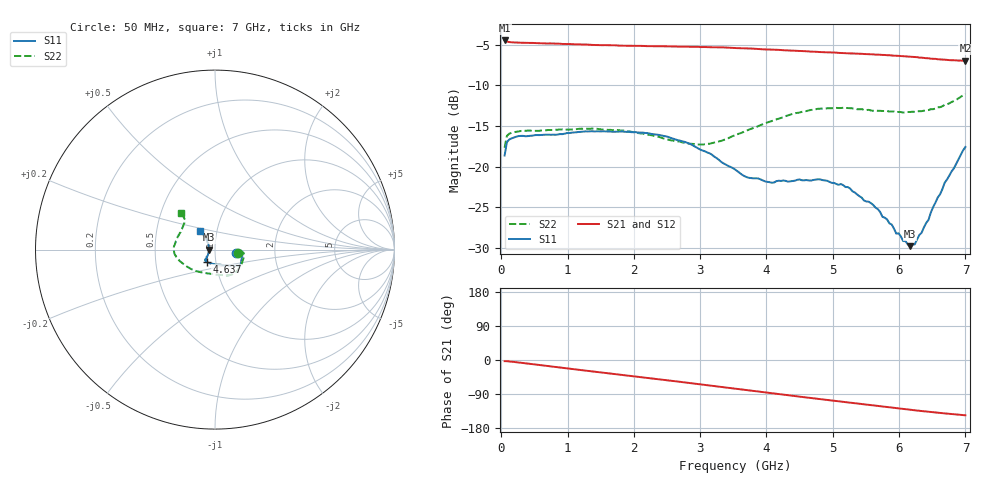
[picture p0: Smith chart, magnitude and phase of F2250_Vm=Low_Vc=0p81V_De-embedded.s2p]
! Integrated Device Technology
! Corporate Headquarters
! 6024 Silver Creek Valley Road
! San Jose, CA 95138  USA
! Phone:  1-408-284-8200
! Toll Free:  1-800-223-1366
! Webpage:  http://www.idt.com/
! Timing and RF Division
! 515 Groton Road, Suite 102
! Westford, MA 01886-6024
! Device:  F2250
! Description: Voltage Variable RF Attenuator
! Frequency:  50.0 -  6000.00 MHz
! Package:  3x3 mm Thin QFN Plastic Package: 16 pin
! Ports:  2 RF, 3 DC
!  Pin  1  = GND
!  Pin  2  = NC
!  Pin  3  = RF1  = Port 1
!  Pin  4  = NC
!  Pin  5  = GND
!  Pin  6  = GND
!  Pin  7  = GND
!  Pin  8  = GND
!  Pin  9  = NC
!  Pin 10  = RF2  = Port 2
!  Pin 11  = NC
!  Pin 12  = GND
!  Pin 13  = GND
!  Pin 14  = VCNTRL
!  Pin 15  = VDD
!  Pin 16  = VMODE
! Vcntrl:  0.810 Volts
! Vmode:  +0.000 Volts
! Vdd:  +3.30  Volts
! Current:  1.166 mA
! Data:  The device was measured on a the F2250 evaluation board which has
!  individual transmission lines to the RF pins.  Data was collected
!  using a calibrated network analyzer.  The evaluation board was
!  de-embedded using a TRL calibration technique.
!  The reference plane is the edge of the package pin.
! Misc:  SN 10
!  Action Tracker AT0258
! Date Measured:  2014-11-26
! Date:  2015-10-15  MJV
! Note:
!  Integrated Device Technology supplies this data as a sample of measured
!  data at the package pin for this product.  Your particular data for this
!  product may vary.
!  Data was taken at 25 degrees C.
!  Integrated Device Technology reserves the right to change this data at anytime.
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# GHz S dB R 50
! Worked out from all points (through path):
!   201 points, 50 MHz to 7 GHz, reference 50 ohm
!   highest |S21| = -4.46 dB at 50 MHz (marker M1); lowest = -7.0 dB at 7 GHz (marker M2)
!   group delay of S21, straight-line fit = 58.5 ps
!   lowest |S11| = -29.8 dB at 6.166 GHz (marker M3), VSWR 1.07, Z = 46.9 - j0.0792 ohm
!   |S11| at or under -10 dB: start of sweep to end of sweep
!   |S22| runs from -17.7 to -11.1 dB; largest |S21 - S12| = 0.0014
!   S11 on the Smith chart (normalised r, x): 50 MHz: 1.26, -0.05; 4.637 GHz: 0.90, -0.12; 7 GHz: 0.83, +0.17
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0.05  -18.64 -8.9  -4.46 -3.0  -4.48 -3.0  -17.67 -8.8
0.08475  -17.00 -5.7  -4.60 -3.2  -4.61 -3.2  -16.22 -6.2
0.22375  -16.32 -6.9  -4.72 -5.7  -4.73 -5.7  -15.72 -9.6
1.2315  -15.70 -27.8  -4.97 -27.2  -4.95 -27.2  -15.33 -43.2
1.857  -15.71 -32.8  -5.12 -40.1  -5.11 -40.1  -15.57 -57.5
2.37825  -16.10 -35.2  -5.17 -50.9  -5.19 -50.9  -16.35 -70.2
3.0385  -18.03 -44.8  -5.28 -65.0  -5.27 -65.0  -17.29 -100.4
3.525  -20.36 -64.6  -5.39 -75.6  -5.41 -75.6  -16.15 -128.5
3.69875  -21.30 -75.4  -5.44 -79.5  -5.45 -79.5  -15.58 -137.1
4.081  -21.99 -100.1  -5.59 -87.7  -5.59 -87.7  -14.39 -154.0
4.637  -21.71 -124.7  -5.82 -99.6  -5.82 -99.6  -13.09 -170.9
4.7065  -21.65 -127.4  -5.85 -101.0  -5.84 -101.0  -13.01 -172.3
5.22775  -22.53 -135.0  -6.06 -111.9  -6.04 -111.9  -12.79 175.9
5.61  -24.73 -138.6  -6.18 -119.8  -6.19 -119.8  -13.13 166.6
5.85325  -26.99 -147.4  -6.28 -124.8  -6.30 -124.8  -13.23 160.1
5.9575  -28.26 -154.3  -6.35 -126.9  -6.36 -126.9  -13.29 157.2
5.99225  -28.22 -157.9  -6.37 -127.7  -6.37 -127.7  -13.27 156.2
6.166  -29.81 -178.5  -6.46 -131.2  -6.47 -131.2  -13.28 150.4
6.2355  -29.59 166.9  -6.51 -132.6  -6.51 -132.7  -13.26 147.8
6.33975  -28.15 151.7  -6.59 -134.7  -6.60 -134.7  -13.17 144.3
6.68725  -22.00 129.0  -6.84 -140.9  -6.86 -140.9  -12.40 134.9
7  -17.59 129.8  -6.96 -146.0  -6.97 -146.0  -11.05 132.5
